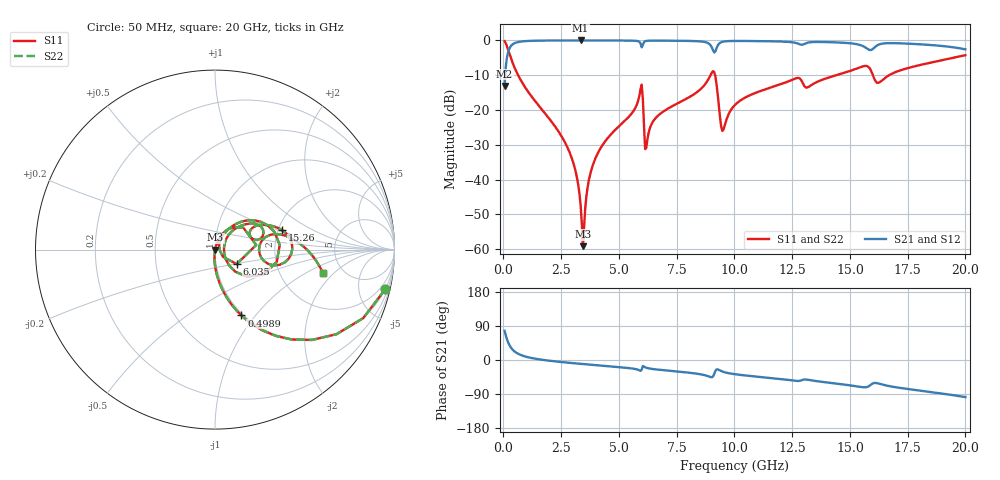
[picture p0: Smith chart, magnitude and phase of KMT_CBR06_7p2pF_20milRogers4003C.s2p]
! Data measured by Modelithics Inc. support@modelithics.com 813-866-6335
! KEMET CBR0603 7.2pF, Pad Width= 0.851mm, Pad Length= 0.64mm, Pad Gap= 0.62mm, 20mil Rogers 4003C substrate Data, January 2022
# hz S ma R 50
! 2 Port Network Data from SP1.SP block
! freq  magS11  angS11  magS21  angS21  magS12  angS12  magS22  angS22
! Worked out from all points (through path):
!   401 points, 50 MHz to 20 GHz, reference 50 ohm
!   highest |S21| = -0.01 dB at 3.342 GHz (marker M1); lowest = -13.1 dB at 50 MHz (marker M2)
!   group delay of S21, straight-line fit = 14.4 ps
!   lowest |S11| = -59.1 dB at 3.442 GHz (marker M3), VSWR 1.00, Z = 50.1 - j0.035 ohm
!   |S11| at or under -10 dB: 635.9 MHz to 8.964 GHz (8.328 GHz wide, 174 % of centre); 9.162 GHz to 14.41 GHz (5.248 GHz wide, 44.5 % of centre); 15.99 GHz to 16.7 GHz (702 MHz wide, 4.29 % of centre)
!   |S22| runs from -59.1 to -0.2 dB; largest |S21 - S12| = 0
!   S11 on the Smith chart (normalised r, x): 50 MHz: 0.98, -8.66; 498.9 MHz: 0.98, -0.85; 6.035 GHz: 1.26, -0.21; 15.26 GHz: 2.11, +0.53; 20 GHz: 3.53, -1.47
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5e7  0.9749 -13.0  0.2225 77.0  0.2225 77.0  0.9749 -13.0
2.495e8  0.6577 -49.6  0.7527 40.3  0.7527 40.3  0.6577 -49.6
4.98875e8  0.3952 -68.2  0.918 21.7  0.918 21.7  0.3952 -68.2
2.74325e9  0.03033 -94.9  0.9985 -6.8  0.9985 -6.8  0.03033 -94.9
3.14225e9  0.01237 -94.2  0.9988 -9.0  0.9988 -9.0  0.01237 -94.2
3.34175e9  0.004252 -85.4  0.9988 -10.1  0.9988 -10.1  0.004252 -85.4
3.391625e9  0.002383 -73.2  0.9988 -10.4  0.9988 -10.4  0.002383 -73.2
3.4415e9  0.001107 -18.4  0.9988 -10.7  0.9988 -10.7  0.001107 -18.4
3.74075e9  0.01136 71.9  0.9987 -12.2  0.9987 -12.2  0.01136 71.9
4.13975e9  0.02597 72.9  0.9983 -14.3  0.9983 -14.3  0.02597 72.9
5.885375e9  0.1611 50.6  0.9533 -27.2  0.9533 -27.2  0.1611 50.6
6.035e9  0.1452 -33.6  0.8603 -16.1  0.8603 -16.1  0.1452 -33.6
6.2345e9  0.03831 51.7  0.988 -21.4  0.988 -21.4  0.03831 51.7
6.73325e9  0.0854 62.3  0.9931 -25.7  0.9931 -25.7  0.0854 62.3
9.0275e9  0.3465 16.1  0.7871 -45.5  0.7871 -45.5  0.3465 16.1
9.476375e9  0.05012 -3.5  0.9547 -30.4  0.9547 -30.4  0.05012 -3.5
1.0025e10  0.1185 47.5  0.9824 -37.5  0.9824 -37.5  0.1185 47.5
1.336662e10  0.2323 29.6  0.9469 -54.1  0.9469 -54.1  0.2323 29.6
1.526188e10  0.3904 15.9  0.8877 -69.2  0.8877 -69.2  0.3904 15.9
1.596012e10  0.3387 -15.0  0.7403 -62.9  0.7403 -62.9  0.3387 -15.0
1.670825e10  0.3179 14.9  0.9141 -69.0  0.9141 -69.0  0.3179 14.9
2e10  0.614 -12.2  0.7439 -97.9  0.7439 -97.9  0.614 -12.2
